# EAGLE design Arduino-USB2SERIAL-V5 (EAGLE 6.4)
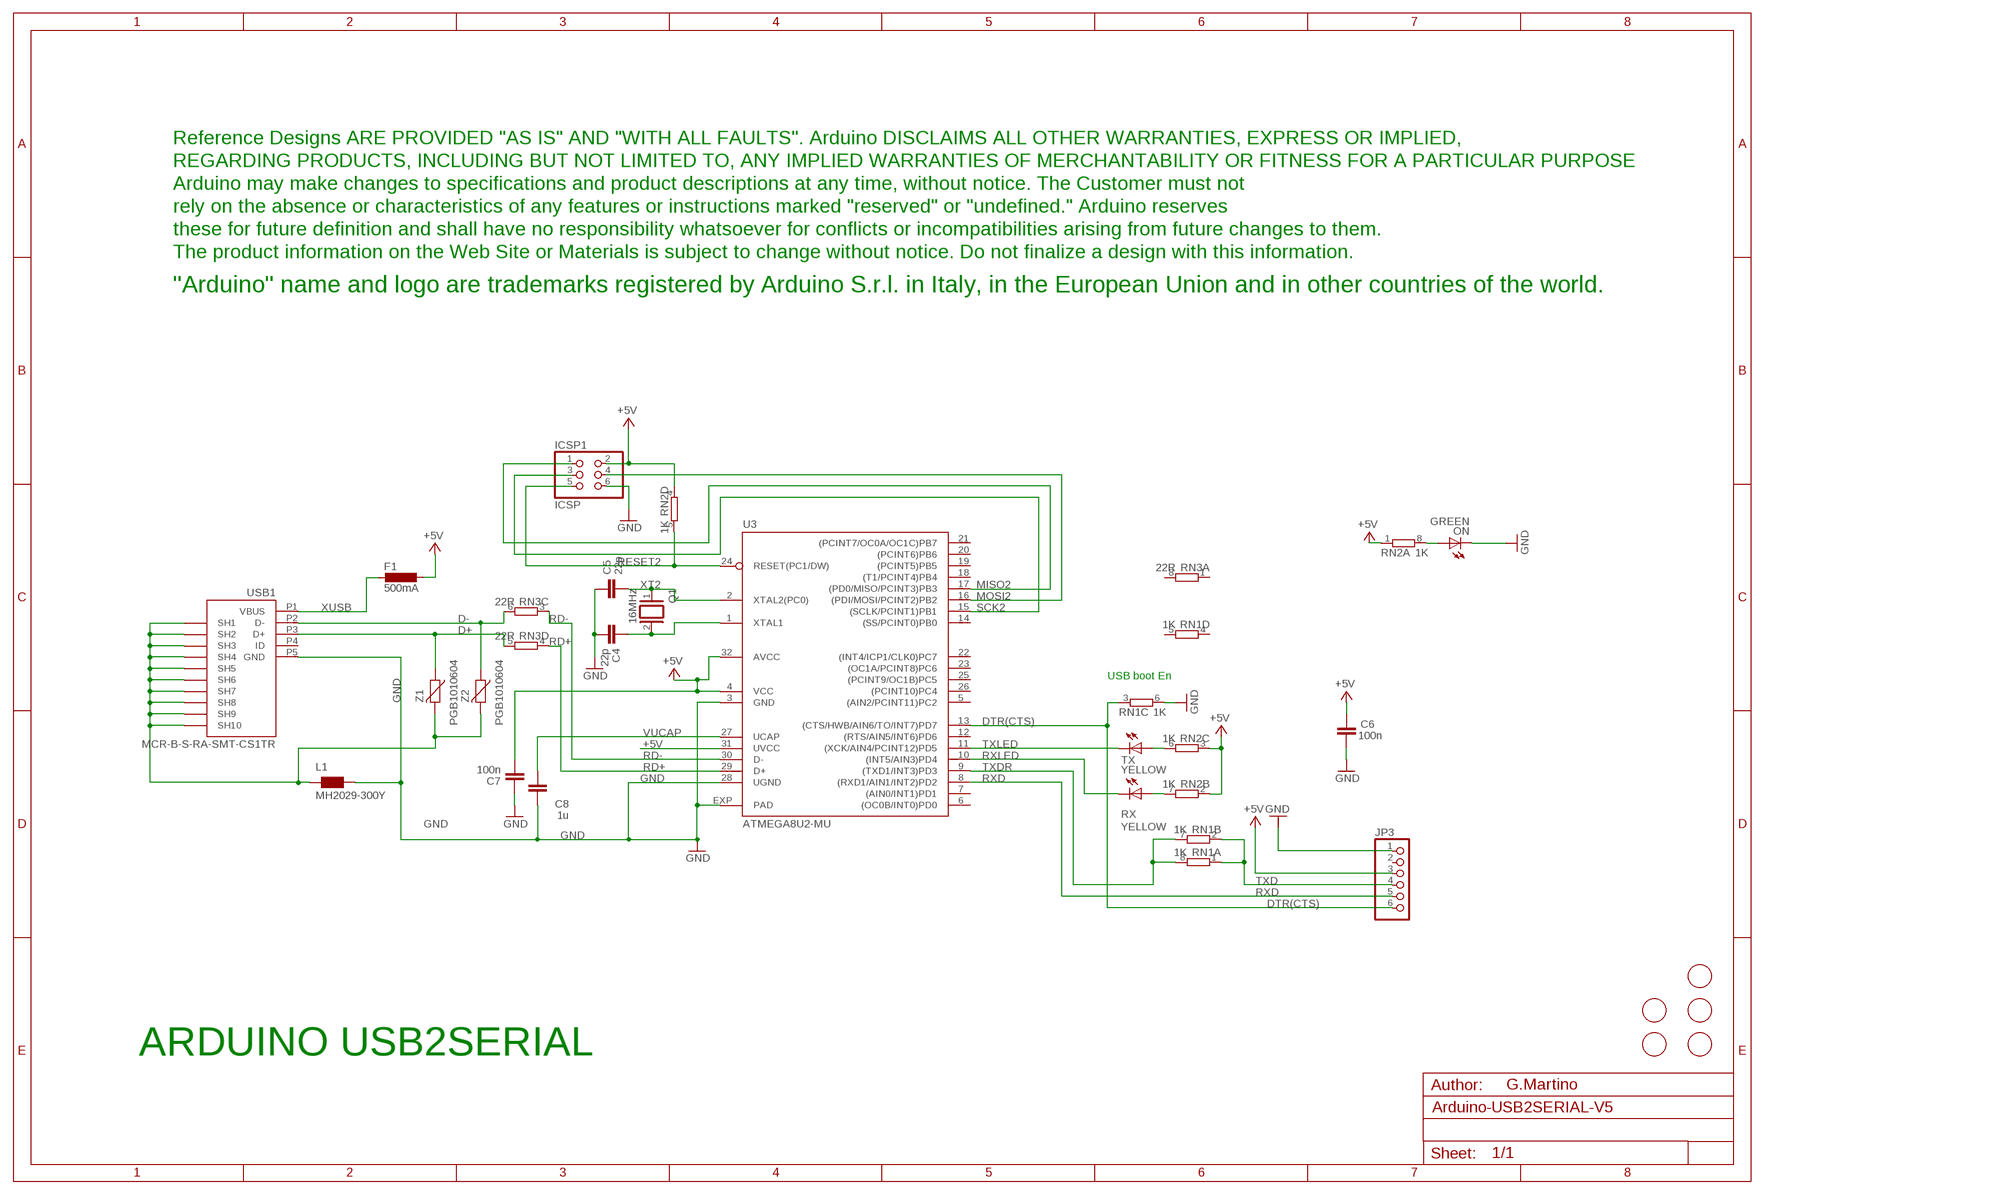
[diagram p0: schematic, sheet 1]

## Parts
C4  22p  C-EU0603-RND  [C0603-ROUND]
C5  22p  C-EU0603-RND  [C0603-ROUND]
C6  100n  C-EU0603-RND  [C0603-ROUND]
C7  100n  C-EU0603-RND  [C0603-ROUND]
C8  1u  C-EU0603-RND  [C0603-ROUND]
F1  500mA  L-EUL1812  [L1812]
ICSP1  ICSP  PINHD-2X3  [2X03]
JP3  PINHD-1X6LITTLE  [1X06_LITTLE]
L1  MH2029-300Y  0001_BLM21PG300SN1D_/_MH2029-300Y  [0805]
ON  GREEN  LEDCHIP-LED0805  [CHIP-LED0805]
Q1  16MHz  XTAL/S  [QS]
RN1  1K  4R-NCAY16  [CAY16]
RN2  1K  4R-NCAY16  [CAY16]
RN3  22R  4R-NCAY16  [CAY16]
RX  YELLOW  LEDCHIP-LED0805  [CHIP-LED0805]
TX  YELLOW  LEDCHIP-LED0805  [CHIP-LED0805]
U3  ATMEGA8U2-MU  [QFN32]
U$1  FIDUCIALMOUNT  [FIDUCIA-MOUNT]
U$2  FIDUCIALMOUNT  [FIDUCIA-MOUNT]
U$3  FIDUCIALMOUNT  [FIDUCIA-MOUNT]
U$4  FIDUCIALMOUNT  [FIDUCIA-MOUNT]
U$6  FIDUCIALMOUNT  [FIDUCIA-MOUNT]
U$7  DISCLAIMER  [DISCLAIMER]
USB1  MCR-B-S-RA-SMT-CS1TR  0158_MCR-B-S-RA-SMT-CS1TR  [CON2_USB_MICRO_B_AT]
Z1  PGB1010604  VARISTORCN0603  [CT/CN0603]
Z2  PGB1010604  VARISTORCN0603  [CT/CN0603]

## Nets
+5V [usbvcc]: C6.2 C7.1 F1.1 ICSP1.2 JP3.3 RN2.1 RN2.2 RN2.3 RN2.4 U3.4(VCC) U3.31(UVCC) U3.32(AVCC)
D+: RN3.5 USB1.P3(D+) Z1.1
D-: RN3.6 USB1.P2(D-) Z2.1
DTR(CTS): JP3.6 RN1.3 U3.13((CTS/HWB/AIN6/TO/INT7)PD7)
GND [gnd]: C4.1 C5.2 C6.1 C7.2 C8.2 ICSP1.6 JP3.1 L1.2 ON.C RN1.6 U3.3(GND) U3.28(UGND) U3.EXP(PAD) USB1.P5(GND)
MISO2: ICSP1.1 U3.17((PD0/MISO/PCINT3)PB3)
MOSI2: ICSP1.4 U3.16((PDI/MOSI/PCINT2)PB2)
N$1: C4.2 Q1.2 U3.1(XTAL1)
N$2: ON.A RN2.8
N$4 [gnd]: L1.1 USB1.P$1(SH7) USB1.P$2(SH8) USB1.P$3(SH9) USB1.P$4(SH10) USB1.P$5(SH7) USB1.P$6(SH8) USB1.P$7(SH9) USB1.P$8(SH10) USB1.S1(SH1) USB1.S2(SH2) USB1.S3(SH3) USB1.S4(SH4) USB1.S5(SH5) USB1.S6(SH6) Z1.2 Z2.2
N$35: RN2.7 RX.A
N$36: RN2.6 TX.A
RD+: RN3.4 U3.29(D+)
RD-: RN3.3 U3.30(D-)
RESET2: ICSP1.5 RN2.5 U3.24(RESET(PC1/DW))
RXD: JP3.5 U3.8((RXD1/AIN1/INT2)PD2)
RXLED: RX.C U3.10((INT5/AIN3)PD4)
SCK2: ICSP1.3 U3.15((SCLK/PCINT1)PB1)
TXD: JP3.4 RN1.1 RN1.2
TXDR: RN1.7 RN1.8 U3.9((TXD1/INT3)PD3)
TXLED: TX.C U3.11((XCK/AIN4/PCINT12)PD5)
VUCAP: C8.1 U3.27(UCAP)
XT2: C5.1 Q1.1 U3.2(XTAL2(PC0))
XUSB [usbvcc]: F1.2 USB1.P1(VBUS)
Unconnected: JP3.2 RN1.4 RN1.5 RN3.1 RN3.2 RN3.7 RN3.8 U3.5((AIN2/PCINT11)PC2) U3.6((OC0B/INT0)PD0) U3.7((AIN0/INT1)PD1) U3.12((RTS/AIN5/INT6)PD6) U3.14((SS/PCINT0)PB0) U3.18((T1/PCINT4)PB4) U3.19((PCINT5)PB5) U3.20((PCINT6)PB6) U3.21((PCINT7/OC0A/OC1C)PB7) U3.22((INT4/ICP1/CLK0)PC7) U3.23((OC1A/PCINT8)PC6) U3.25((PCINT9/OC1B)PC5) U3.26((PCINT10)PC4) USB1.P4(ID)

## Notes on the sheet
- USB boot En
- ARDUINO USB2SERIAL
- G.Martino

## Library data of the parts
C4-C8 = SmartPrj:C-EU: CAPACITOR, European symbol
F1 = rcl:L-EU: INDUCTOR, European symbol
ICSP1 = pinhead:PINHD-2X3: PIN HEADER
JP3 = SmartPrj:PINHD-1X6: PIN HEADER
L1 = Protezione:0001_BLM21PG300SN1D_/_MH2029-300Y: BLM21; MONTHLY_USAGE: _____; PART_NUMBER: BLM21PG300SN1D_/_MH2029-300Y; PRICE: _____; SUPPLIER: _____; TYPE: Protezione
ON RX TX = led:LED: LED
Q1 = special:XTAL/S: CRYSTAL
RN1-RN3 = resistor-dil:4R-N: Array Chip Resistor Source: RS Component / Phycomp
U3 = atmel:ATMEGA8U2-MU
U$1-U$4 U$6 = SmartPrj:FIDUCIALMOUNT
U$7 = Misc:DISCLAIMER
USB1 = Connettori:0158_MCR-B-S-RA-SMT-CS1TR: Usb Micro F/90 Smd Tipo B; MONTHLY_USAGE: _____; PART_NUMBER: MCR-B-S-RA-SMT-CS1TR; PRICE: _____; SUPPLIER: _____; TYPE: Connettori
Z1 Z2 = varistor:VARISTOR: VARISTOR

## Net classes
0 default: width 0.254 mm, clearance 0.254 mm
1 power: width 0.61 mm, clearance 0.254 mm
2 gnd: width 0.305 mm, drill 0.559 mm, clearance 0.254 mm
3 usbvcc: width 0.356 mm, clearance 0.254 mm
4 aref: width 0.406 mm, drill 0.61 mm, clearance 0.254 mm

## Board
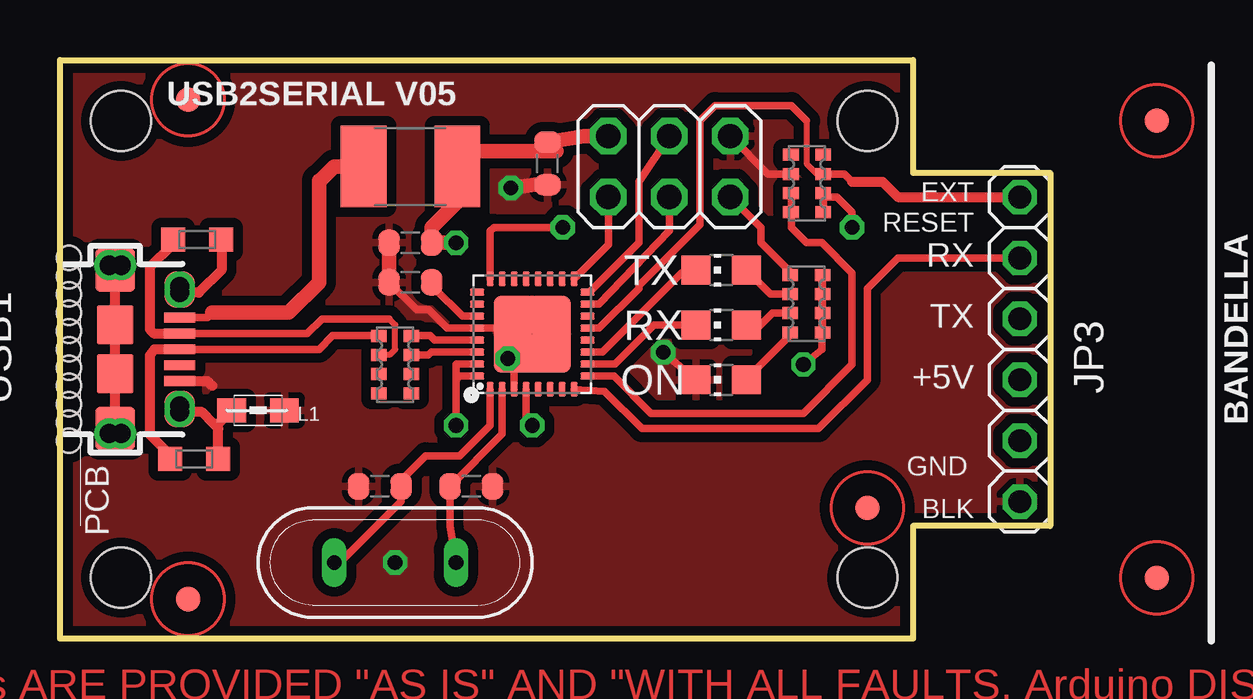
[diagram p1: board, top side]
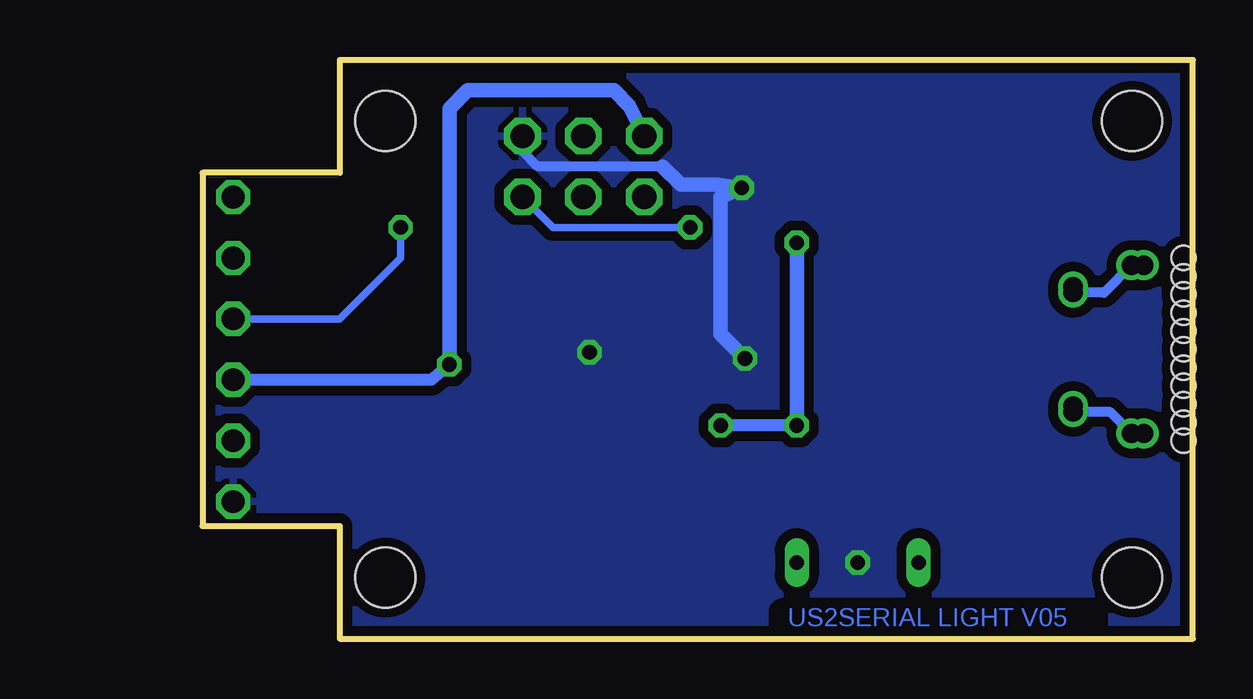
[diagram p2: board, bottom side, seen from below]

Size 41.27 x 24.13 mm. Coordinates in mm from the lower left corner, seen from the top.
Outline: 0,0 0,24.13 35.56,24.13 35.56,19.43 41.27,19.43 41.27,4.7 35.56,4.7 35.56,0 0,0
Copper layers (1*16): Top 0.035mm / dielectric 1.5mm / Bottom 0.035mm
Design rules "ArduinoDEF *": minimum track width 6mil, minimum drill 12mil, track to track 5mil, track to pad 5mil, pad to pad 5mil, via to via 5mil, smd to smd 4mil, copper to edge 10mil, drill to drill 6mil, minimum pad ring 8mil, minimum via ring 8mil, stop-mask expansion 0mil, vias tented up to drill 24mil, thermal gap 10mil
Holes 2.5 mm at 2.54,21.59 2.54,2.54 33.66,2.54 33.66,21.59
Holes 1 mm at 0.38,15.88 0.38,15.11 0.38,14.35 0.38,13.59 0.38,12.83 0.38,12.06 0.38,11.3 0.38,10.54 0.38,9.78 0.38,9.02 0.38,8.26
bRestrict: 4 lines

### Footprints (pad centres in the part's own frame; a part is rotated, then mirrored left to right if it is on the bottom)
C0603-ROUND = smd 0.898 x 1.1: 1 -0.889,0; 2 0.889,0
L1812 = smd 1.9 x 3.4: 1 -1.95,0; 2 1.95,0
2X03 = drill 1.016 octagon: 1 -2.54,-1.27; 2 -2.54,1.27; 3 0,-1.27; 4 0,1.27; 5 2.54,-1.27; 6 2.54,1.27
1X06_LITTLE = drill 0.95 pad 1.422 octagon: 1 -6.35,0; 2 -3.81,0; 3 -1.27,0; 4 1.27,0; 5 3.81,0; 6 6.35,0
0805 = smd 1.2 x 1: 1 -1.1,0; 2 1.1,0
CHIP-LED0805 = smd 1.2 x 1.2: A 0,-1.05; C 0,1.05
QS = drill 0.61 long: 1 -2.54,0; 2 2.54,0
CAY16 = smd 0.5 x 0.65: 1 -1.2,-0.675; 2 -0.4,-0.675; 3 0.4,-0.675; 4 1.2,-0.675; 5 1.2,0.675; 6 0.4,0.675; 7 -0.4,0.675; 8 -1.2,0.675
QFN32 = smd 0.6 x 0.3: 1 -2.3,1.75; 2 -2.3,1.25; 3 -2.3,0.75; 4 -2.3,0.25; 5 -2.3,-0.25; 6 -2.3,-0.75; 7 -2.3,-1.25; 8 -2.3,-1.75; 17 2.3,-1.75; 18 2.3,-1.25; 19 2.3,-0.75; 20 2.3,-0.25; 21 2.3,0.25; 22 2.3,0.75; 23 2.3,1.25; 24 2.3,1.75 | smd 0.3 x 0.6: 9 -1.75,-2.3; 10 -1.25,-2.3; 11 -0.75,-2.3; 12 -0.25,-2.3; 13 0.25,-2.3; 14 0.75,-2.3; 15 1.25,-2.3; 16 1.75,-2.3; 25 1.75,2.3; 26 1.25,2.3; 27 0.75,2.3; 28 0.25,2.3; 29 -0.25,2.3; 30 -0.75,2.3; 31 -1.25,2.3; 32 -1.75,2.3 | smd 3.2 x 3.2: EXP 0,0
FIDUCIA-MOUNT = smd 1.016 x 1.016: P$1 0,0
FIDUCIA-MOUNT@1 = smd 1.016 x 1.016: P$1 0,0
CON2_USB_MICRO_B_AT = smd 0.406 x 1.346: P1 -1.321,2.692; P2 -0.66,2.692; P3 0,2.692; P4 0.66,2.692; P5 1.321,2.692 | drill 0.8 pad 1.24: P$1 -2.616,2.692; P$2 -2.362,2.692; P$7 2.362,2.692; P$8 2.616,2.692 | drill 0.8 pad 1.25: P$3 -3.505,-0.254; P$4 -3.505,0.254; P$5 3.505,0.254; P$6 3.505,-0.254 | smd 1.778 x 1.651: S1 -3.302,0; S2 3.302,0 | smd 1.524 x 1.27: S3 -2.489,2.692; S4 2.489,2.692 | smd 1.626 x 1.524: S5 -1.016,0; S6 1.016,0
CT/CN0603 = smd 1 x 1: 1 -1,0; 2 1,0

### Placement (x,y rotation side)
C4  13.34,6.35 0 top
C5  17.14,6.35 0 top
C6  20.32,19.81 90 top
C7  14.61,16.51 180 top
C8  14.61,14.86 180 top
F1  14.61,19.68 180 top
ICSP1  25.4,19.68 0 top
JP3  40.01,12.06 90 top
L1  8.26,9.53 0 top
ON  27.56,10.79 90 top
Q1  13.97,3.17 180 top
RN1  31.14,18.98 90 top
RN2  31.11,13.97 90 top
RN3  13.97,11.43 90 top
RX  27.56,13.08 90 top
TX  27.56,15.37 90 top
U3  19.68,12.7 90 top
U$1  5.33,22.48 0 top
U$2  5.33,1.65 0 top
U$3  FIDUCIALMOUNT  [FIDUCIA-MOUNT@1]  33.66,5.46 0 top
U$4  FIDUCIALMOUNT  [FIDUCIA-MOUNT@1]  not placed on the board
U$6  FIDUCIALMOUNT  [FIDUCIA-MOUNT@1]  not placed on the board
U$7  not placed on the board
USB1  2.3,12.06 270 top
Z1  5.59,7.49 0 top
Z2  5.71,16.64 0 top

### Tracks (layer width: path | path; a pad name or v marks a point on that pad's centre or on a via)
+5V  (via drill 0.61)
  Top 0.305: RN2.1 RN2.2 RN2.3 RN2.4 31.75,15.21 31.75,12.06 v30.99,11.43 | v16.51,8.89 16.51,10.79 | 16.51,10.79 16.51,11.43 16.53,11.45 U3.31 | U3.32 16.66,10.95 16.51,10.79 | U3.4 19.43,9.14 v19.68,8.89
  Top 0.61: ICSP1.2 21.84,20.95 C6.2 20.7,20.32 17.14,20.32 F1.1 16.55,18.21 15.49,17.14 C7.1 v16.51,16.51
  Bottom 0.508: v16.51,8.89 v19.68,8.89 | v30.99,11.43 31.75,10.79 JP3.3
  Bottom 0.61: ICSP1.2 23.5,22.23 24.13,22.86 30.23,22.86 30.99,22.1 v30.99,11.43 | v16.51,8.89 v16.51,16.51
D+
  Top 0.305: RN3.5 11.36,12.63 10.79,12.06 USB1.P3
  Top 0.406: USB1.P3 3.94,12.06 3.75,11.81 3.75,8.51 4.59,7.67 Z1.1
D-
  Top 0.254: RN3.6 13.73,11.83 13.97,12.06 13.97,13.08 13.72,13.34
  Top 0.305: USB1.P2 10.31,12.72 10.92,13.34 13.72,13.34
  Top 0.406: 4.45,16.64 Z2.1 4.71,16.46 3.75,15.49 3.75,12.89 3.91,12.72 USB1.P2
DTR(CTS)
  Top 0.254: RN1.3 31.55,19.38 31.11,19.81 31.11,21.59
  Top 0.305: U3.13 22.48,12.95 24.13,14.61 24.13,14.73 26.67,17.27 26.67,21.59 27.3,22.23 30.48,22.23 31.11,21.59 | 33.02,19.05 32.69,19.38 RN1.3
  Top 0.406: 33.02,19.05 34.29,19.05 34.92,18.41 JP3.6
GND  (via drill 0.61)  (1 unrouted)
  Top 0.305: v25.15,11.94 ON.C | U3.3 18.93,11.95 U3.EXP 19.43,12.95 U3.28 16.13,12.95 15.37,13.72 14.86,13.72 C8.2 | RN1.6 29.52,19.38 ICSP1.6
  Top 0.406: USB1.P5 6.15,10.74 6.35,10.54
  Top 0.61: C6.1 19.81,18.92 v18.8,18.8 | C8.2 C7.2
  Bottom 0.406: 22.1,19.68 27.3,19.68 27.94,20.32 ICSP1.6
  Bottom 0.61: v18.67,11.68 U3.EXP 19.68,18.41 v18.8,18.8 19.81,18.92 21.34,18.92 22.1,19.68
  other vias: 13.97,3.17
  pour Top (isolate 0.406): 0,24.13 35.56,24.13 35.56,19.68 41.27,19.68 41.27,4.45 35.56,4.45 35.56,0 0,0
  pour Bottom (isolate 0.406): -0.64,24.77 35.56,24.77 35.56,19.68 41.91,19.68 41.91,4.45 36.2,4.45 36.2,-0.64 -0.64,-0.64
MISO2
  Top 0.305: ICSP1.1 22.86,16.43 U3.17
MOSI2
  Top 0.305: U3.16 22.07,14.45 24.13,16.51 24.13,19.05 ICSP1.4
N$1
  Top 0.305: U3.1 17.93,8.89 16.66,7.62 15.24,7.62 14.22,6.6 C4.2 14.22,5.71 11.68,3.17 Q1.2
N$2
  Top 0.305: RN2.8 30.44,12.66 28.57,10.79 ON.A
N$4
  Top 0.406: USB1.S2 USB1.S6 USB1.S5 USB1.S1 | USB1.S1 2.25,15.37 USB1.P$3 | USB1.S1 2.35,15.37 USB1.P$4 | USB1.P$1 USB1.S3 USB1.P$2 5.79,14.43 6.73,15.37 6.73,16.62 Z2.2 | USB1.P$7 USB1.S4 USB1.P$8 5.92,9.45 6.41,8.95 | Z1.2 6.6,7.51 6.6,8.76 6.41,8.95 | L1.1 6.58,8.95 6.41,8.95
  Top 0.61: USB1.P$5 2.5,8.56 USB1.S2 2.1,8.56 USB1.P$6
  Bottom 0.406: USB1.P$4 3.7,14.43 USB1.P$2 | USB1.P$5 3.44,9.45 USB1.P$8
N$35
  Top 0.305: RX.A 28.83,12.7 29.7,13.57 RN2.7
N$36
  Top 0.305: RN2.6 29.61,14.37 TX.A
RD+
  Top 0.305: U3.29 15.62,12.45 15.44,12.63 RN3.4
RD-
  Top 0.305: U3.30 15.48,11.95 15.35,11.83 RN3.3
RESET2  (via drill 0.61)
  Top 0.305: RN2.5 30.44,15.28 29.21,16.51 29.21,17.14 ICSP1.5 | U3.24 17.93,16.99 18.09,17.14 v20.95,17.14
  Bottom 0.305: v20.95,17.14 26.67,17.14 ICSP1.5
RXD
  Top 0.305: U3.8 22.7,10.31 24.26,8.76 31.62,8.76 33.66,10.79 33.66,14.61 34.92,15.88 JP3.5
RXLED
  Top 0.305: U3.10 23.13,11.45 24.77,13.08 RX.C
SCK2
  Top 0.305: U3.15 22.46,13.95 25.4,17.02 ICSP1.3
TXD  (via drill 0.61)
  Top 0.305: v33.02,17.14 33.02,17.78 32.38,18.41 31.98,18.41 RN1.2 RN1.1
  Bottom 0.305: JP3.4 35.56,13.34 33.02,15.88 v33.02,17.14
TXDR
  Top 0.305: U3.9 23.09,10.95 24.64,9.4 30.99,9.4 33.02,11.43 33.02,15.24 31.75,16.51 31.11,16.51 30.48,17.14 RN1.8 | RN1.8 RN1.7 | RN1.8
TXLED
  Top 0.305: U3.11 22.62,11.95 25.91,15.24 TX.C
VUCAP
  Top 0.305: U3.27 16.78,13.45 15.62,14.61 15.62,14.73 C8.1
XT2
  Top 0.305: U3.2 18.43,8.53 C5.1 16.26,4.7 Q1.1
XUSB
  Top 0.305: USB1.P1 6.15,13.39 6.35,13.59
  Top 0.61: F1.2 11.43,19.68 10.84,19.09 10.79,19.09 10.79,14.86 9.53,13.59 6.35,13.59

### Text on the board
Top: ARDUINO USB2SERIAL LIGHT | Reference Designs ARE PROVIDED "AS IS" AND "WITH ALL FAULTS. Arduino DISCLAIMS ALL OTHER WARRANTIES, EXPRESS OR IMPLIED, | REGARDING PRODUCTS, INCLUDING BUT NOT LIMITED TO, ANY IMPLIED WARRANTIES OF MERCHANTABILITY OR FITNESS FOR A PARTICULAR PURPOSE | Arduino may make changes to specifications and product descriptions at any time, without notice. The Customer must not | rely on the absence or characteristics of any features or instructions marked "reserved" or "undefined." Arduino reserves | these for future definition and shall have no responsibility whatsoever for conflicts or incompatibilities arising from future changes to them. | The product information on the Web Site or Materials is subject to change without notice. Do not finalize a design with this information. | ARDUINO is a registered trademark
Bottom: US2SERIAL LIGHT V05
tPlace: USB2SERIAL V05 | EXT | RESET | RX | TX | TX | RX | +5V | BANDELLA | GND | BLK
tNames: Arduino
214bmp: D:/SmartProjects/Snc/a4_bn_logo2.bmp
